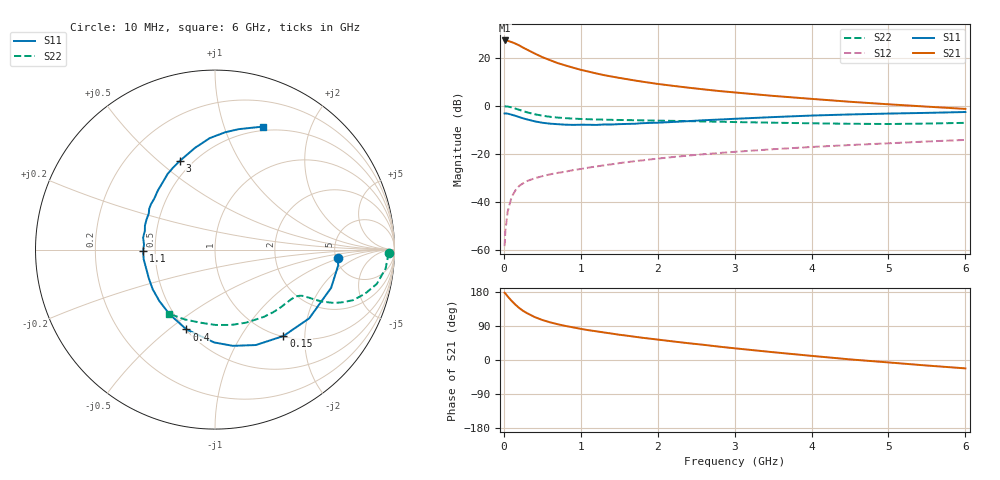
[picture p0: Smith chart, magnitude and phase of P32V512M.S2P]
! SIEMENS Small Signal Semiconductors
! BFP181
! Si NPN RF Bipolar Junction Transistor in SOT143
! VCE = 2.5 V  IC = 12 mA
! Common Emitter S-Parameters:  March  1996
# GHz  S  MA  R  50
!  f  S11  S21  S12  S22
! GHz  MAG  ANG  MAG  ANG  MAG  ANG  MAG  ANG
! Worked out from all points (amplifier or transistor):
!   36 points, 10 MHz to 6 GHz, reference 50 ohm
!   highest |S21| = 27.1 dB at 10 MHz (marker M1)
!   |S21| within 3 dB of that: start of sweep to 251.6 MHz
!   unconditionally stable (mu >= 1): 858.8 MHz to end of sweep
!   at 250 MHz: K = 0.42, MSG = 28.2 dB, |S12| = -32.3 dB
!   at 1.4 GHz: K = 1.19, MAG = 15.6 dB, |S12| = -24.4 dB
!   at 6 GHz: K = 1.02, MAG = 5.7 dB, |S12| = -14.3 dB
!   S11 on the Smith chart (normalised r, x): 10 MHz: 5.22, -0.90; 150 MHz: 1.01, -1.57; 400 MHz: 0.50, -0.58; 1.1 GHz: 0.43, -0.01; 3 GHz: 0.43, +0.59; 6 GHz: 0.46, +1.37
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0.01  0.6865 -3.8  22.62 177.4  0.0012 78.4  0.9686 -1.1
0.02  0.6917 -7.4  22.55 175.4  0.0025 85.6  0.9644 -2.4
0.05  0.6812 -18.2  22.3 167.8  0.0063 86.9  0.9565 -6.3
0.1  0.6498 -36.1  20.96 156.3  0.0125 72.0  0.9212 -12.0
0.15  0.6142 -51.6  19.45 146.1  0.0173 66.9  0.8701 -16.5
0.2  0.5785 -66.8  17.83 137.2  0.0215 62.3  0.8193 -20.1
0.25  0.5453 -79.5  16.06 129.7  0.0243 58.0  0.7697 -22.4
0.3  0.5173 -90.5  14.63 123.8  0.027 55.1  0.7279 -24.1
0.4  0.4722 -109.7  12.14 113.4  0.0309 51.6  0.6633 -25.9
0.5  0.4407 -125.0  10.19 105.6  0.0342 50.0  0.6177 -26.7
0.6  0.4222 -137.3  8.815 99.5  0.0373 50.4  0.5866 -27.1
0.7  0.4114 -147.6  7.662 94.4  0.04 49.8  0.5646 -27.6
0.9  0.3977 -164.4  6.158 86.1  0.0457 50.6  0.5376 -28.6
1.1  0.4005 -178.7  5.098 78.7  0.0515 50.8  0.5215 -30.0
1.5  0.4126 161.1  3.775 66.7  0.0638 51.3  0.5035 -34.1
1.8  0.4316 148.1  3.149 58.7  0.0728 50.8  0.4934 -38.0
2.2  0.4578 134.1  2.578 49.0  0.0855 48.8  0.4822 -43.8
3  0.5324 111.4  1.881 30.9  0.1096 44.0  0.4556 -57.3
3.5  0.5778 101.1  1.594 20.6  0.1242 40.6  0.442 -67.2
4.5  0.6558 85.1  1.203 1.6  0.1516 32.9  0.4198 -89.7
5.5  0.707 73.6  0.953 -14.6  0.1798 25.6  0.4239 -113.3
6  0.7368 68.5  0.855 -22.1  0.1938 21.1  0.4387 -125.3
